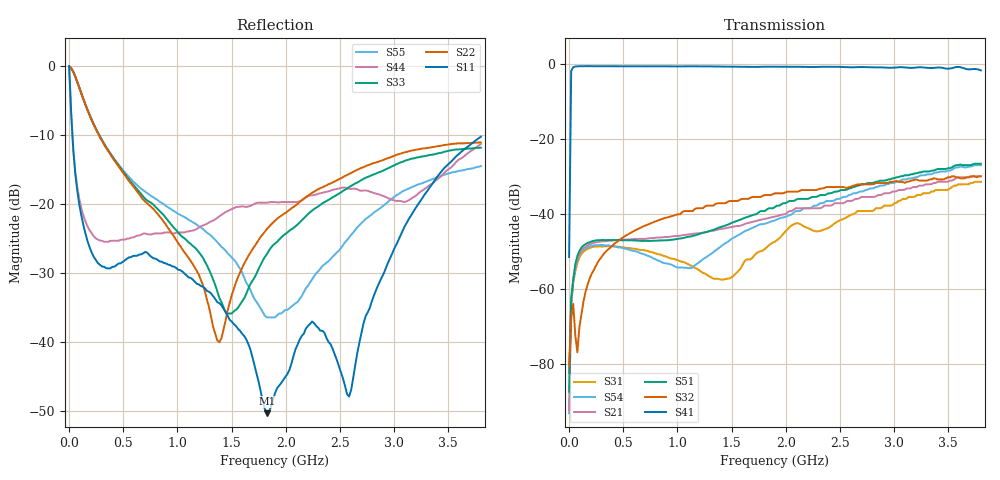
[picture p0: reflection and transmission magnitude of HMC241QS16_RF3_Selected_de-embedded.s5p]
! Hittite Microwave Corporation
! 20 Alpha Road
! Chelmsford, MA 01824
! Tel: 978-250-3343
! Fax: 978-250-3373
! Device: HMC241QS16, DC-3.5 GHz GaAs MMIC SP4T Non-Reflective Switch in 16 lead QSOP package
! Misc: Data was de-embedded to package pins.
!  Port 1 = RFC
!  Port 2 = RF1
!  Port 3 = RF2
!  Port 4 = RF3
!  Port 5 = RF4
!  Vdd  = + 5 V
!  RF3 selected, Vctl= 0/+5 V
!  Data reformated to new Touchstone file format - Tue Jan 09 10:09:53 2007
# MHz S DB R 50
! 5 Port Network Data
! freq  dbS11  angS11  dbS12  angS12  dbS13  angS13  dbS14  angS14
!  dbS15  angS15
!  dbS21  angS21  dbS22  angS22  dbS23  angS23
!  dbS24  angS24  dbS25  angS25
!  dbS31  angS31  dbS32  angS32
!  dbS33  angS33  dbS34  angS34  dbS35  angS35
!  dbS41  angS41
!  dbS42  angS42  dbS43  angS43  dbS44  angS44  dbS45  angS45
!  dbS51  angS51  dbS52  angS52  dbS53  angS53  dbS54  angS54
!  dbS55  angS55
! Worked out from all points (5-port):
!   201 points, 30 kHz to 3.8 GHz, reference 50 ohm
!   strongest paths, dB at 30 kHz, 950 MHz, 1.9 GHz, 2.85 GHz, 3.8 GHz:
!     S41: -51.4, -0.6, -0.7, -0.9, -1.7
!     S32: -80.1, -40.5, -34.4, -31.7, -29.9
!     S51: -87.3, -46.8, -38.1, -31.3, -26.6
!     S21: -92.3, -45.9, -40.6, -34.9, -29.9
!     S54: -93.1, -53.5, -41.6, -32.7, -26.9
!     S31: -82.3, -51.9, -47.3, -38.4, -31.4
!   lowest |S11| = -50.4 dB at 1.824 GHz (marker M1), VSWR 1.01, Z = 49.8 + j0.219 ohm
!   |S11| at or under -10 dB: 30.57 MHz to end of sweep
